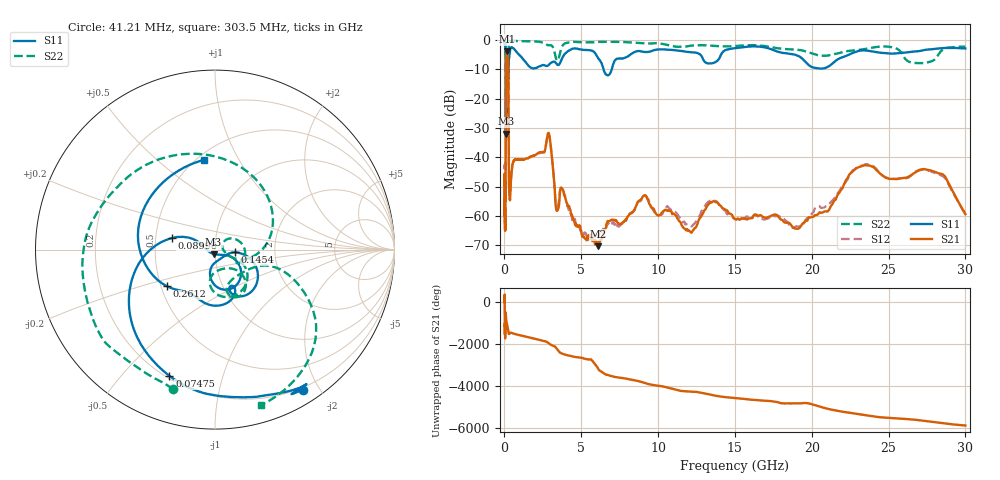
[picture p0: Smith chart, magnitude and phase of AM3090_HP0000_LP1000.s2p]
! Date/Time: Thu, Feb 28, 2019 1:53 PM
! Network Analyzer: Agilent Technologies E8364B Rev: A.07.50.67
! Sweep from 0.010 to 30.000 GHz, 1601 Points, Sweep Type: LOG
! Power Supply: 5.023 V, 0.002 A
# Hz S DB R 50
!freq MagS11 AngS11 MagS21 AngS21 MagS12 AngS12 MagS22 AngS22
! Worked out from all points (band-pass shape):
!   1601 points, 10 MHz to 30 GHz, reference 50 ohm
!   highest |S21| = -3.82 dB at 147.6 MHz (marker M1); lowest = -70.3 dB at 6.11 GHz (marker M2)
!   |S21| within 3 dB of the highest: 99.12 MHz to 238.3 MHz (139.2 MHz wide, 82.5 % of centre)
!   lowest |S11| = -31.9 dB at 97.94 MHz (marker M3), VSWR 1.05, Z = 49.2 - j2.38 ohm
!   |S11| at or under -10 dB: 88.9 MHz to 258.1 MHz (169.2 MHz wide, 97.5 % of centre); 6.454 GHz to 6.981 GHz (526.2 MHz wide, 7.83 % of centre)
!   |S22| runs from -27.4 to -0.1 dB; largest |S21 - S12| = 0.012
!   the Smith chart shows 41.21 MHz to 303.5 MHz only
!   S11 on the Smith chart (normalised r, x): 41.21 MHz: 0.17, -1.79; 74.75 MHz: 0.21, -0.68; 89.96 MHz: 0.61, +0.08; 145.4 MHz: 1.25, -0.04; 261.2 MHz: 0.54, -0.25; 303.5 MHz: 0.54, +0.73
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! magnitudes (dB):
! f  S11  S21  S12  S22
! 10 MHz  -0.2  -49.5  -44.0  -0.6
! 38.04 MHz  -0.5  -59.0  -59.8  -1.5
! 41.21 MHz  -0.7  -63.9  -61.8  -1.8
! 74.75 MHz  -2.5  -44.6  -44.6  -4.6
! 89.96 MHz  -12.0  -14.4  -14.3  -11.4
! 97.94 MHz  -31.9  -7.2  -7.2  -26.0
! 114.4 MHz  -12.8  -4.8  -4.8  -17.5
! 144.7 MHz  -19.9  -3.8  -3.8  -16.5
! 145.4 MHz  -19.1  -3.8  -3.8  -16.4
! 147.6 MHz  -17.0  -3.8  -3.8  -15.9
! 232.8 MHz  -10.3  -6.3  -6.2  -10.7
! 261.2 MHz  -9.5  -15.2  -15.1  -9.7
! 303.5 MHz  -5.9  -50.4  -50.3  -0.9
! 550.5 MHz  -2.7  -42.0  -42.0  -0.2
! 2.084 GHz  -9.5  -38.9  -39.0  -0.5
! 2.884 GHz  -8.5  -31.8  -31.8  -1.7
! 3.419 GHz  -8.3  -58.2  -56.9  -7.0
! 6.11 GHz  -6.2  -70.3  -66.8  -0.6
! 7.926 GHz  -5.9  -61.2  -61.6  -0.7
! 18.93 GHz  -5.0  -64.3  -63.6  -3.3
! 23.48 GHz  -3.5  -42.6  -42.3  -3.0
! 30 GHz  -2.8  -59.3  -59.3  -2.2
